(* Logix 5000 AddOnInstructionDefinition export AMCI_NXFE2_Resume; software revision 20.03 *)

ADD_ON_INSTRUCTION AMCI_NXFE2_Resume   (* revision 1.0, vendor AMCI *)
VAR_IN_OUT
   NXFE2_output_data : _000A:NXFE2_0986AEB4:O:0; {required}
END_VAR
VAR
   command_data_block : INT[10];
        [0]   // Command Bits MSW
        [1]   // Command Bits LSW
        [2]   // Upper Target Position
        [3]   // Lower Target Position
        [4]   // Upper Programmed Speed
        [5]   // Lower Programmed Speed
END_VAR

ROUTINE Logic   (* ladder *)
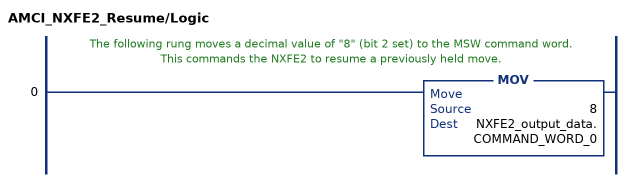
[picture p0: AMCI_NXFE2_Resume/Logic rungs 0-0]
   // The following rung moves a decimal value of "8" (bit 2 set) to the MSW command word.  This commands the NXFE2 to resume a previously held move.
   0: MOV(8,NXFE2_output_data.COMMAND_WORD_0);
END_ROUTINE
END_ADD_ON_INSTRUCTION
